(* Logix 5000 AddOnInstructionDefinition export AMCI_SD4840E2_Immediate_Stop; software revision 20.03 *)

ADD_ON_INSTRUCTION AMCI_SD4840E2_Immediate_Stop   (* revision 1.0, vendor AMCI *)
VAR_IN_OUT
   AMCI_SD4840E2_output_data : _000A:SD4840E2_4342D302:O:0; {required}
END_VAR
VAR
   command_data_block : INT[10];
        [0]   // Command Bits MSW
        [1]   // Command Bits LSW
        [2]   // Upper Target Position
        [3]   // Lower Target Position
        [4]   // Upper Programmed Speed
        [5]   // Lower Programmed Speed
END_VAR

ROUTINE Logic   (* ladder *)
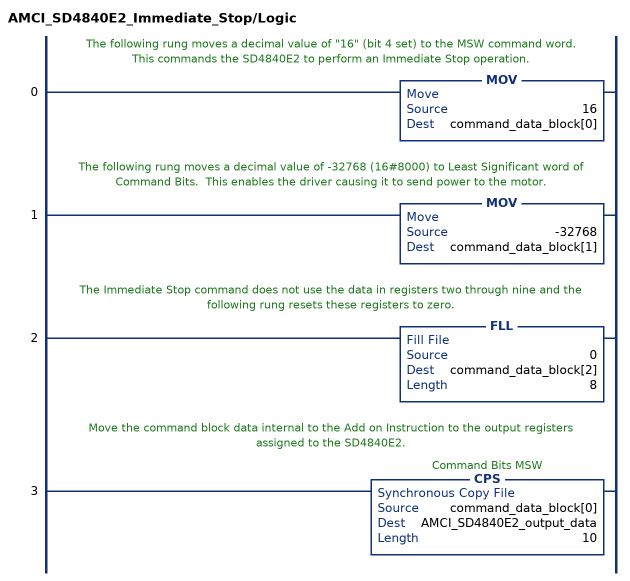
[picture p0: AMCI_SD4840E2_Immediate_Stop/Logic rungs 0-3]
   // The following rung moves a decimal value of "16" (bit 4 set) to the MSW command word.  This commands the SD4840E2 to perform an Immediate Stop operation.
   0: MOV(16,command_data_block[0]);
   // The following rung moves a decimal value of -32768 (16#8000) to Least Significant word of Command Bits.  This enables the driver causing it to send power to the motor.
   1: MOV(-32768,command_data_block[1]);
   // The Immediate Stop command does not use the data in registers two through nine and the following rung resets these registers to zero.
   2: FLL(0,command_data_block[2],8);
   // Move the command block data internal to the Add on Instruction to the output registers assigned to the SD4840E2.
   3: CPS(command_data_block[0],AMCI_SD4840E2_output_data,10);
END_ROUTINE
END_ADD_ON_INSTRUCTION
